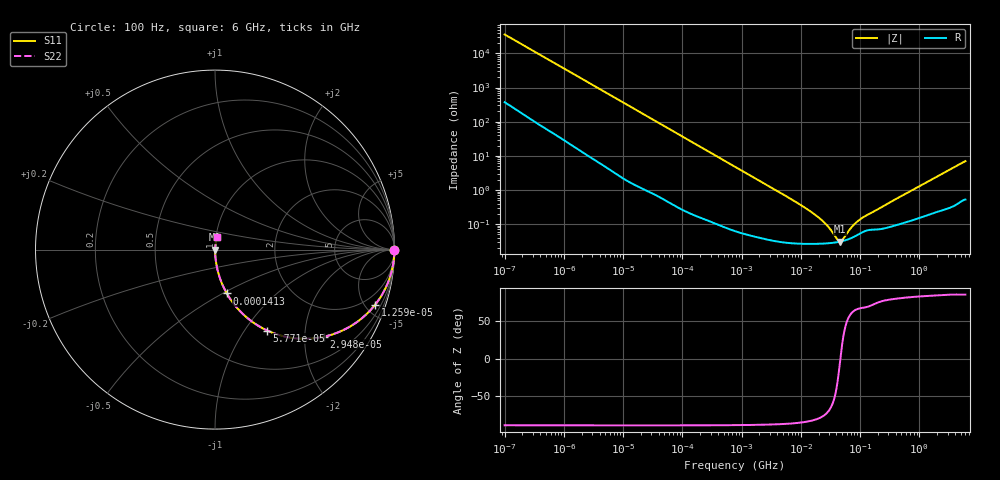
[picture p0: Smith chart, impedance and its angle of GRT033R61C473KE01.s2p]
!Murata Part Number: GRT033R61C473KE01
!These Parameters are Measured in Series Mode Connection
!Data Generated on Jun 19, 2026
!  o--ll--o
!Port1  Port2
!  o------o
!Operation Temp=25[degC], DC Bias Voltage=0[V]
!Freq. Start=100[Hz] Stop=6[GHz] 401[Steps]
# Hz S RI R 50
!Freq.(Hz) S11(Real) S11(Imag) S21(Real) S21(Imag) S12(Real) S12(Imag) S22(Real) S22(Imag)
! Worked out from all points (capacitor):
!   401 points, 100 Hz to 6 GHz, reference 50 ohm
!   read as one part in series: C = 44.4 nF near 109 Hz
!   lowest |Z| = 30.8 mohm at 45.56 MHz (marker M1)
!   series resonance near 46.59 MHz, so ESL is about 260 pH
!   S11 on the Smith chart (normalised r, x): 100 Hz: open; 12.59 kHz: 1.03, -5.82; 29.48 kHz: 1.02, -2.49; 57.71 kHz: 1.01, -1.28; 141.3 kHz: 1.00, -0.52; 6 GHz: 1.01, +0.14
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100  1 -0.0028  3.69e-05 0.0028  3.69e-05 0.0028  1 -0.0028
2008  0.9966 -0.055  0.00344 0.055  0.00344 0.055  0.9966 -0.055
5378  0.9779 -0.1439  0.0221 0.1439  0.0221 0.1439  0.9779 -0.1439
12592  0.8929 -0.3063  0.1071 0.3063  0.1071 0.3063  0.8929 -0.3063
18841  0.7897 -0.4044  0.2103 0.4044  0.2103 0.4044  0.7897 -0.4044
29482  0.6076 -0.485  0.3924 0.485  0.3924 0.485  0.6076 -0.485
40335  0.4545 -0.4945  0.5455 0.4945  0.5455 0.4945  0.4545 -0.4945
57709  0.291 -0.4508  0.709 0.4508  0.709 0.4508  0.291 -0.4508
90302  0.1449 -0.3486  0.8551 0.3486  0.8551 0.3486  0.1449 -0.3486
141303  0.0657 -0.244  0.9343 0.244  0.9343 0.244  0.0657 -0.244
302498  0.0159 -0.1205  0.9841 0.1205  0.9841 0.1205  0.0159 -0.1205
774597  0.00293 -0.0479  0.9971 0.0479  0.9971 0.0479  0.00293 -0.0479
6353432  0.000312 -0.00582  0.9997 0.00582  0.9997 0.00582  0.000312 -0.00582
1.555665e7  0.000267 -0.00215  0.9997 0.00215  0.9997 0.00215  0.000267 -0.00215
2.545746e7  0.000271 -0.00104  0.9997 0.00104  0.9997 0.00104  0.000271 -0.00104
4.165952e7  0.000297 -0.00018  0.9997 0.00018  0.9997 0.00018  0.000297 -0.00018
4.556224e7  0.000305 -3.53e-05  0.9997 3.53e-05  0.9997 3.53e-05  0.000305 -3.53e-05
4.983056e7  0.000316 0.000108  0.9997 -0.000108  0.9997 -0.000108  0.000316 0.000108
7.129496e7  0.00039 0.000693  0.9996 -0.000693  0.9996 -0.000693  0.00039 0.000693
9.753859e7  0.000517 0.00122  0.9995 -0.00122  0.9995 -0.00122  0.000517 0.00122
3.124326e8  0.00083 0.00416  0.9992 -0.00416  0.9992 -0.00416  0.00083 0.00416
6e9  0.00993 0.0684  0.9901 -0.0684  0.9901 -0.0684  0.00993 0.0684
